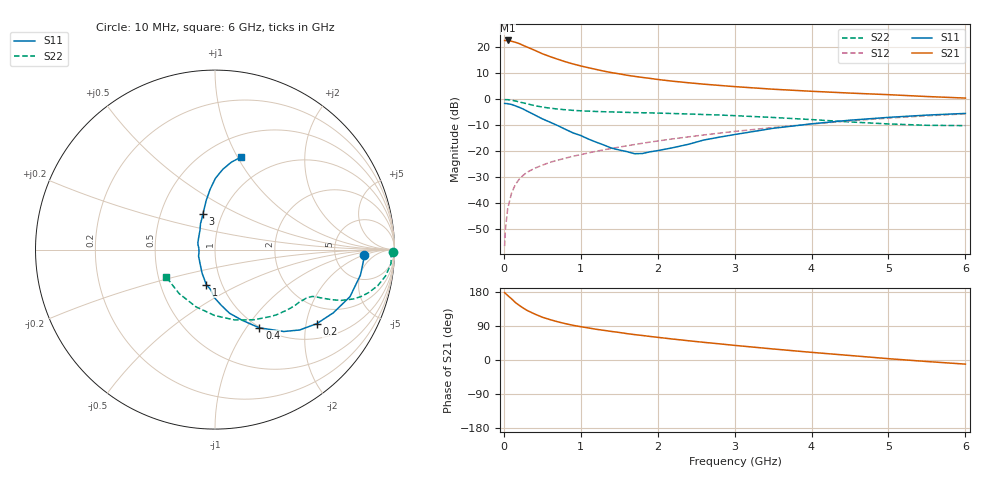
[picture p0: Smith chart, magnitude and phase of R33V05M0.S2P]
! SIEMENS Small Signal Semiconductors
! BFR181
! Si NPN RF Bipolar Junction Transistor in SOT23
! VCE = 3 V  IC = 5 mA
! Common Emitter S-Parameters:  May  1996
# GHz  S  MA  R  50
!  f  S11  S21  S12  S22
! GHz  MAG  ANG  MAG  ANG  MAG  ANG  MAG  ANG
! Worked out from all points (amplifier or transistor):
!   36 points, 10 MHz to 6 GHz, reference 50 ohm
!   highest |S21| = 22.6 dB at 50 MHz (marker M1)
!   |S21| within 3 dB of that: start of sweep to 338.9 MHz
!   unconditionally stable (mu >= 1): 1.115 GHz to 2.951 GHz
!   at 250 MHz: K = 0.42, MSG = 25.0 dB, |S12| = -29.3 dB
!   at 1.4 GHz: K = 1.05, MAG = 13.3 dB, |S12| = -18.9 dB
!   at 6 GHz: K = 0.86, MSG = 3.0 dB, |S12| = -5.6 dB
!   lowest NFmin = 1.55 dB at 450 MHz
!   S11 on the Smith chart (normalised r, x): 10 MHz: 11, -2; 200 MHz: 1.42, -2.30; 400 MHz: 0.99, -1.15; 1 GHz: 0.84, -0.34; 3 GHz: 0.81, +0.34; 6 GHz: 0.72, +1.03
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0.01  0.833 -2.0  13.5 178.0  0.0015 91.2  0.9916 -0.9
0.02  0.8304 -3.9  13.47 175.9  0.0031 86.4  0.9815 -1.8
0.05  0.8228 -9.9  13.53 170.3  0.0079 84.6  0.9837 -4.6
0.1  0.7966 -19.2  13.05 161.4  0.0157 81.9  0.9616 -8.8
0.15  0.7475 -28.1  12.48 151.8  0.023 75.3  0.9287 -12.5
0.2  0.7009 -36.1  11.77 144.2  0.0291 72.3  0.8908 -15.5
0.25  0.6505 -43.5  10.9 137.3  0.0344 68.8  0.8551 -17.8
0.3  0.5957 -50.0  10.13 131.1  0.0395 67.1  0.8197 -19.6
0.4  0.5013 -60.4  8.767 121.4  0.0471 64.5  0.7561 -22.0
0.5  0.421 -69.1  7.518 112.9  0.0541 63.7  0.7083 -23.2
0.6  0.3632 -77.2  6.625 106.6  0.0614 63.2  0.6756 -23.9
0.7  0.3122 -83.6  5.896 100.9  0.0675 63.2  0.6488 -24.5
0.8  0.2648 -91.3  5.27 95.9  0.0737 63.0  0.6294 -24.9
1  0.2011 -104.1  4.377 87.9  0.0863 63.7  0.6003 -25.8
1.1  0.1718 -110.8  4.045 84.6  0.0932 64.0  0.5916 -26.5
1.6  0.0985 -158.4  2.901 69.6  0.1275 64.3  0.5604 -30.7
2.2  0.1174 139.6  2.223 55.2  0.1736 62.8  0.5326 -37.7
3  0.21 108.6  1.753 38.6  0.2409 58.1  0.4846 -50.3
3.5  0.2767 100.3  1.562 29.1  0.2865 54.1  0.4474 -60.9
4.5  0.3965 89.7  1.316 11.9  0.3849 43.9  0.367 -90.4
5.5  0.4966 79.3  1.13 -4.0  0.4814 31.2  0.3163 -129.3
6  0.5351 74.3  1.055 -10.9  0.5252 24.1  0.3117 -150.9
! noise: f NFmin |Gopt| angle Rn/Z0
0.45  1.55  0.48  17  0.36
0.9  1.65  0.4  35  0.34
1.8  2  0.18  88  0.34
